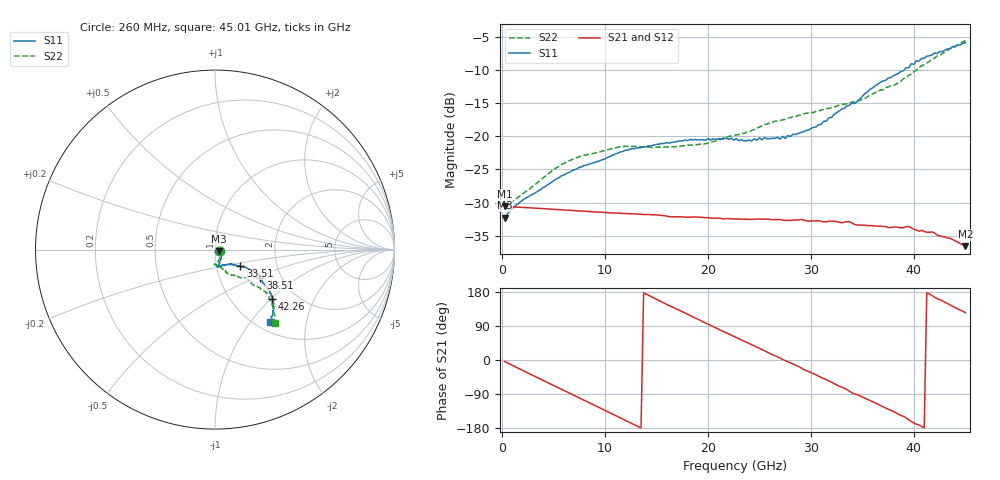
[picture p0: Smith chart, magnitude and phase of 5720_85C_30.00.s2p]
! Device:  ADRF5720
! Description: 0.5dB LSB GaAs MMIC 6-bit Digital Attenuator
! Frequency:  0.000009 -  40 GHz
! Ports:
!	RF1	= Port 1
!	RF2	= Port 2
! Vdd:  3.3 Volt
! Vss:  -3.3 Volt
! Control:  0/3.3 Volt
! State:  30.00 dB attenuation
! Data:  The device was measured using G-S-G Probes on a matrix board.
!  Data was collected using an calibrated 4 port network analyzer.
!  The reference plane for this measurement is at the launchers.
! Note:  Analog Devices supplies this data as a sample of measured data
!  for this product.  Your particular data for this product may vary.
!  Data was taken at 85 degrees C.
!  Analog Devices reserves the right to change this data at anytime.
# GHZ S DB R 45.0
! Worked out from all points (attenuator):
!   180 points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, 260 MHz to 45.01 GHz, reference 45 ohm
!   highest |S21| = -30.59 dB at 260 MHz (marker M1); lowest = -36.6 dB at 45.01 GHz (marker M2)
!   lowest |S11| = -32.3 dB at 260 MHz (marker M3), VSWR 1.05, Z = 47.1 - j0.735 ohm
!   |S11| at or under -10 dB: start of sweep to 39.08 GHz
!   |S22| runs from -31.2 to -5.6 dB; largest |S21 - S12| = 0.00022
!   S11 on the Smith chart (normalised r, x): 260 MHz: 1.05, -0.02; 33.51 GHz: 1.30, -0.25; 38.51 GHz: 1.57, -0.54; 42.26 GHz: 1.51, -1.02; 45.01 GHz: 1.15, -1.26
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0.26  -32.26 -18.6  -30.59 -3.7  -30.59 -3.7  -31.18 -17.8
1.76  -29.92 -5.0  -30.72 -24.1  -30.71 -24.1  -28.98 -18.1
5.01  -26.73 -38.4  -31.02 -67.2  -31.01 -67.1  -25.06 -62.0
7.76  -24.62 -53.9  -31.29 -103.4  -31.28 -103.3  -22.98 -78.3
11.51  -22.39 -70.2  -31.63 -152.7  -31.62 -152.6  -21.60 -91.5
15.26  -21.21 -78.8  -31.91 156.8  -31.90 156.9  -21.66 -92.6
19.51  -20.51 -82.1  -32.27 101.1  -32.26 101.3  -21.21 -81.8
22.76  -20.36 -77.8  -32.49 59.2  -32.47 59.5  -19.81 -72.6
24.26  -20.72 -74.4  -32.54 40.6  -32.53 40.8  -19.13 -69.4
25.51  -20.19 -69.3  -32.50 24.3  -32.48 24.5  -18.24 -68.1
27.51  -20.33 -60.8  -32.70 -1.3  -32.68 -1.1  -17.47 -63.6
30.26  -18.65 -45.6  -32.75 -36.1  -32.73 -35.9  -16.45 -61.7
33.51  -15.40 -33.2  -32.88 -78.3  -32.86 -77.9  -15.09 -54.5
34.26  -15.09 -34.1  -33.32 -89.5  -33.31 -89.3  -14.84 -52.2
35.76  -12.92 -29.8  -33.48 -107.1  -33.47 -106.8  -13.78 -49.1
37.76  -11.19 -29.5  -33.78 -132.8  -33.77 -132.2  -12.39 -42.6
38.51  -10.54 -31.6  -33.75 -143.1  -33.72 -142.8  -11.93 -41.9
39.51  -9.69 -34.6  -33.63 -157.8  -33.62 -157.5  -10.78 -42.6
40.26  -8.62 -36.9  -34.16 -169.4  -34.14 -168.9  -10.06 -41.1
42.26  -7.53 -41.1  -34.91 161.9  -34.89 162.2  -7.92 -41.2
43.51  -6.79 -43.9  -35.39 145.5  -35.38 145.7  -6.80 -45.1
45.01  -5.88 -53.0  -36.58 125.0  -36.52 125.3  -5.57 -50.5
